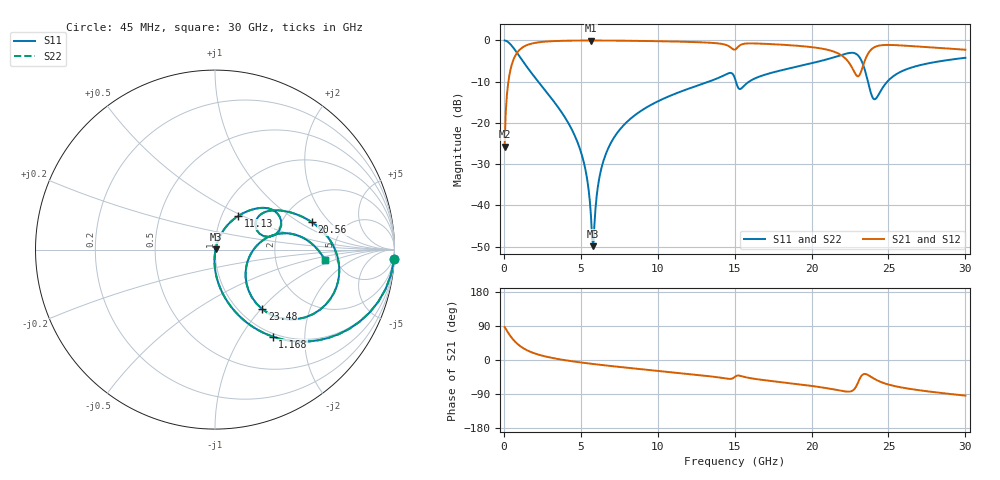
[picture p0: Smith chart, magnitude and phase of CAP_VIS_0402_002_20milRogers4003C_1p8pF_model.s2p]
! S-parameter model data by Modelithics Inc.  support@modelithics.com  813-866-6335  Tampa FL USA
! S-Parameter data specifications:
! Substrate: 20-mil Rogers 4003C, substrate thickness, H=0.508mm, Dielectric constant, Er=3.75
! PCB Mounting Pad Footprint: Pad width, PadW=0.50mm , Pad length, PadL=0.50mm , Pad gap, PadG (edge-to-edge)=0.40mm , Reference planes=1.4mm apart
! Created Wed Nov 18 12:43:11 2015
# hz S ma R 50
! 2 Port Network Data from SP1.SP block
! freq  magS11  angS11  magS21  angS21  magS12  angS12  magS22  angS22
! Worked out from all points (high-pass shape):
!   401 points, 45 MHz to 30 GHz, reference 50 ohm
!   highest |S21| = -0.03 dB at 5.662 GHz (marker M1); lowest = -25.8 dB at 45 MHz (marker M2)
!   |S21| within 3 dB of the highest: 852.6 MHz to 21.65 GHz (20.8 GHz wide, 185 % of centre); 23.7 GHz to end of sweep
!   lowest |S11| = -49.9 dB at 5.811 GHz (marker M3), VSWR 1.01, Z = 50.3 + j0.0697 ohm
!   |S11| at or under -10 dB: 2.231 GHz to 13.31 GHz (11.08 GHz wide, 143 % of centre); 15.08 GHz to 15.93 GHz (848.4 MHz wide, 5.47 % of centre); 23.67 GHz to 24.92 GHz (1.255 GHz wide, 5.17 % of centre)
!   |S22| runs from -49.9 to 0.0 dB; largest |S21 - S12| = 0
!   S11 on the Smith chart (normalised r, x): 45 MHz: 1, -38; 1.168 GHz: 0.95, -1.40; 11.13 GHz: 1.19, +0.47; 20.56 GHz: 2.92, +1.30; 23.48 GHz: 1.26, -1.02; 30 GHz: 4.05, -0.76
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4.5e7  0.9987 -3.0  0.05153 87.0  0.05153 87.0  0.9987 -3.0
4.194375e8  0.9002 -26.6  0.4351 63.4  0.4351 63.4  0.9002 -26.6
1.168312e9  0.582 -56.4  0.812 33.5  0.812 33.5  0.582 -56.4
2.4414e9  0.2823 -77.7  0.9574 12.0  0.9574 12.0  0.2823 -77.7
5.062462e9  0.04112 -93.0  0.9963 -6.8  0.9963 -6.8  0.04112 -93.0
5.4369e9  0.01939 -90.3  0.9968 -8.8  0.9968 -8.8  0.01939 -90.3
5.661562e9  0.007365 -76.5  0.9969 -9.9  0.9969 -9.9  0.007365 -76.5
5.811338e9  0.003215 12.4  0.9969 -10.6  0.9969 -10.6  0.003215 12.4
6.260662e9  0.02446 70.0  0.9964 -12.7  0.9964 -12.7  0.02446 70.0
6.93465e9  0.05645 70.9  0.9949 -15.8  0.9949 -15.8  0.05645 70.9
1.007992e10  0.1856 59.7  0.978 -29.0  0.978 -29.0  0.1856 59.7
1.112835e10  0.2258 55.6  0.969 -33.2  0.969 -33.2  0.2258 55.6
1.50225e10  0.3441 13.7  0.7731 -44.2  0.7731 -44.2  0.3441 13.7
1.539694e10  0.2593 28.8  0.8843 -42.1  0.8843 -42.1  0.2593 28.8
2.003996e10  0.5311 19.3  0.8272 -68.6  0.8272 -68.6  0.5311 19.3
2.056418e10  0.5615 15.7  0.8014 -71.7  0.8014 -71.7  0.5615 15.7
2.258614e10  0.7082 -14.7  0.4846 -82.3  0.4846 -82.3  0.7082 -14.7
2.303546e10  0.6541 -33.4  0.367 -58.1  0.367 -58.1  0.6541 -33.4
2.348479e10  0.425 -51.6  0.5823 -36.9  0.5823 -36.9  0.425 -51.6
2.408389e10  0.1931 -19.7  0.8273 -49.8  0.8273 -49.8  0.1931 -19.7
2.505742e10  0.3359 14.0  0.8813 -65.4  0.8813 -65.4  0.3359 14.0
3e10  0.6158 -5.4  0.7715 -94.0  0.7715 -94.0  0.6158 -5.4
